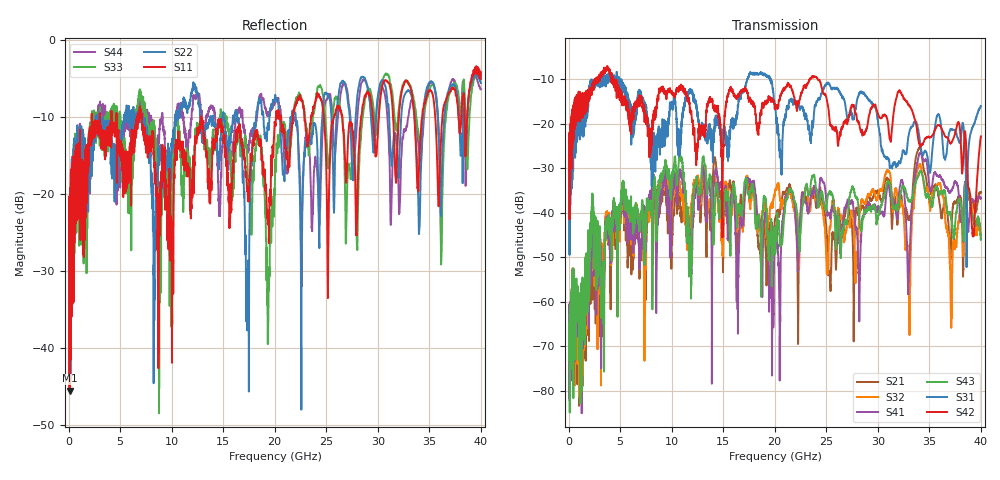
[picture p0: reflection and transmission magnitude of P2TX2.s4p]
!Agilent Technologies,N5245A,MY49151084,A.09.20.08
!Agilent N5245A: A.09.20.08
!Date: Thursday, March 01, 2012 14:03:24
!Correction: S11(Full 4 Port(1,2,3,4))
!S12(Full 4 Port(1,2,3,4))
!S13(Full 4 Port(1,2,3,4))
!S14(Full 4 Port(1,2,3,4))
!S21(Full 4 Port(1,2,3,4))
!S22(Full 4 Port(1,2,3,4))
!S23(Full 4 Port(1,2,3,4))
!S24(Full 4 Port(1,2,3,4))
!S31(Full 4 Port(1,2,3,4))
!S32(Full 4 Port(1,2,3,4))
!S33(Full 4 Port(1,2,3,4))
!S34(Full 4 Port(1,2,3,4))
!S41(Full 4 Port(1,2,3,4))
!S42(Full 4 Port(1,2,3,4))
!S43(Full 4 Port(1,2,3,4))
!S44(Full 4 Port(1,2,3,4))
!S4P File: Measurements: <S11,S12,S13,S14>,
!<S21,S22,S23,S24>,
!<S31,S32,S33,S34>,
!<S41,S42,S43,S44>:
# Hz S  dB  R 50
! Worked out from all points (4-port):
!   3996 points, 50 MHz to 40 GHz, reference 50 ohm
!   strongest paths, dB at 50 MHz, 10.04 GHz, 20.03 GHz, 30.02 GHz, 40 GHz:
!     S42: -26.4, -13.0, -16.5, -17.8, -22.8
!     S31: -24.7, -15.2, -15.5, -19.5, -16.0
!     S43: -64.8, -32.2, -49.3, -40.9, -45.7
!     S41: -68.5, -37.4, -45.0, -38.5, -36.8
!     S32: -62.8, -40.1, -35.0, -36.2, -44.9
!     S21: -66.5, -47.2, -41.5, -35.1, -35.4
!   lowest |S11| = -45.6 dB at 90 MHz (marker M1), VSWR 1.01, Z = 50.1 + j0.519 ohm
!   |S11| at or under -10 dB: start of sweep to 2.239 GHz; 7.076 GHz to 12.85 GHz (5.773 GHz wide, 57.9 % of centre); 12.85 GHz to 20.12 GHz (7.267 GHz wide, 44.1 % of centre)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
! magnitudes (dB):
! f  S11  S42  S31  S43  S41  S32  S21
! 50 MHz  -21.9  -26.4  -24.7  -64.8  -68.5  -62.8  -66.5
! 90 MHz  -45.6  -41.5  -49.4  -72.2  -81.8  -69.4  -70.8
! 10.85 GHz  -14.3  -12.0  -22.7  -27.1  -30.3  -34.7  -38.6
! 17.33 GHz  -19.2  -13.0  -9.9  -34.1  -32.8  -32.2  -31.6
! 19.72 GHz  -17.2  -14.2  -10.4  -56.5  -62.9  -37.8  -43.3
! 21.46 GHz  -15.0  -11.7  -14.6  -34.8  -35.1  -35.0  -33.7
! 40 GHz  -5.1  -22.8  -16.0  -45.7  -36.8  -44.9  -35.4
